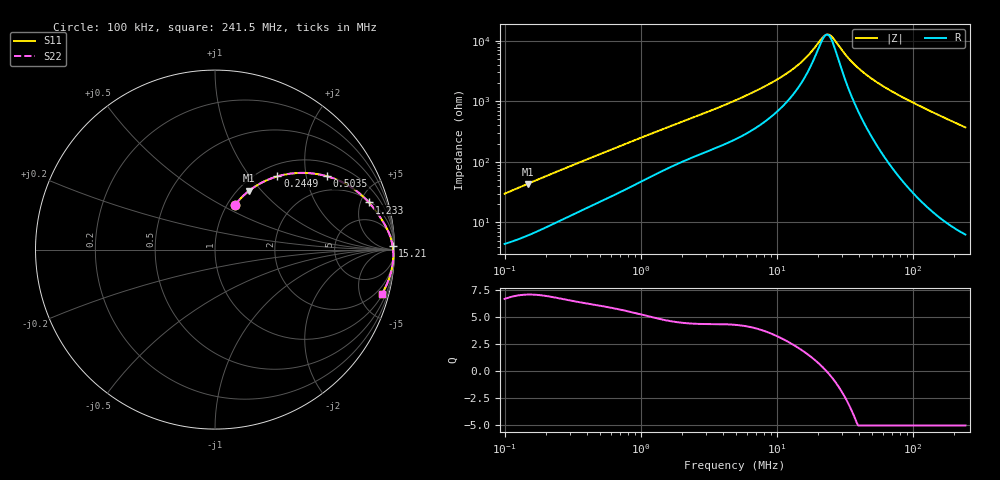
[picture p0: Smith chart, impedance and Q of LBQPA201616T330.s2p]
! LBQPA201616T330  S-PARAMETER MODEL  ( General Type )
! Model Generated by TAIYO YUDEN Corporation (http://www.ty-top.com)
! Version 1.0
! TAIYO YUDEN Control No. 191025NI43SB-FBB
! Copyright(c) 2019 TAIYO YUDEN CO.,LTD. All Rights Reserved.
! Product Description (link to TY-COMPAS)
! https://ds.yuden.co.jp/TYCOMPAS/or/detail?pn=LBQPA201616T330K&u=M
! Products Name : Inductors
! Characteristics :
!  Inductance : 33 uH , SRF(min) : 14 MHz , DC Resistance(max) : 3.64 Ohm
!  Rated Current : Saturation :220 mA , Temp Rise : 165 mA (20 degC)
!  Case Size : 2.0 x 1.6 / 0.079 x 0.063 [mm/inch] , Thickness : 1.6 / 0.063 [mm/inch]
!  (Conditions: Temperature = 25 degC , DC Bias Current/Voltage = 0A / 0V)
! External Node Assignments :
!  1  o---GGG---o  2
! GND o---------o GND
! Frequency Range : 0.1MHz  -  241.513628MHz  [ 402 STEP ]
# MHz S RI R 50
! Freq[MHz].  S11 Real  S11 Imag  S21 Real  S21 Imag  S12 Real  S12 Imag  S22 Real  S22 Imag
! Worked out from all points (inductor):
!   401 points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, 100 kHz to 241.5 MHz, reference 50 ohm
!   read as one part in series: L = 46.5 uH near 104 kHz
!   highest Q = 7.07 at 147.6 kHz (marker M1), where L = 46.2 uH
!   self-resonance near 22.89 MHz
!   S11 on the Smith chart (normalised r, x): 100 kHz: 1.09, +0.59; 244.9 kHz: 1.20, +1.38; 503.5 kHz: 1.44, +2.65; 1.233 MHz: 2.19, +5.89; 15.21 MHz: 42, +80; 241.5 MHz: 1.13, -7.40
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0.1  0.1128 0.2502  0.8872 -0.2502  0.8872 -0.2502  0.1128 0.2502
0.147621  0.1897 0.3277  0.8103 -0.3277  0.8103 -0.3277  0.1897 0.3277
0.244928  0.3479 0.408  0.6521 -0.408  0.6521 -0.408  0.3479 0.408
0.368674  0.5058 0.4272  0.4942 -0.4272  0.4942 -0.4272  0.5058 0.4272
0.503455  0.6244 0.4085  0.3756 -0.4085  0.3756 -0.4085  0.6244 0.4085
0.787915  0.7652 0.3433  0.2348 -0.3433  0.2348 -0.3433  0.7652 0.3433
1.233101  0.8578 0.2626  0.1422 -0.2626  0.1422 -0.2626  0.8578 0.2626
1.359207  0.8723 0.2459  0.1277 -0.2459  0.1277 -0.2459  0.8723 0.2459
4.914404  0.97 0.09  0.03 -0.09  0.03 -0.09  0.97 0.09
9.715792  0.9852 0.0424  0.0148 -0.0424  0.0148 -0.0424  0.9852 0.0424
12.5148  0.9879 0.0289  0.0121 -0.0289  0.0121 -0.0289  0.9879 0.0289
15.20538  0.9895 0.0194  0.0105 -0.0194  0.0105 -0.0194  0.9895 0.0194
18.11814  0.9907 0.0112  0.00925 -0.0112  0.00925 -0.0112  0.9907 0.0112
22.0134  0.9919 0.00227  0.00813 -0.00227  0.00813 -0.00227  0.9919 0.00227
24.26464  0.9924 -0.00227  0.00764 0.00227  0.00764 0.00227  0.9924 -0.00227
25.72444  0.9926 -0.00505  0.00737 0.00505  0.00737 0.00505  0.9926 -0.00505
32.49632  0.9935 -0.0167  0.00652 0.0167  0.00652 0.0167  0.9935 -0.0167
38.72134  0.9938 -0.0263  0.00619 0.0263  0.00619 0.0263  0.9938 -0.0263
48.91461  0.9937 -0.0408  0.00634 0.0408  0.00634 0.0408  0.9937 -0.0408
66.79689  0.992 -0.0641  0.00801 0.0641  0.00801 0.0641  0.992 -0.0641
119.8055  0.9804 -0.1264  0.0196 0.1264  0.0196 0.1264  0.9804 -0.1264
241.5136  0.9284 -0.2495  0.0716 0.2495  0.0716 0.2495  0.9284 -0.2495
